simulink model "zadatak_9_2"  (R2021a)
settings: Solver=VariableStepAuto  StartTime=0.0  StopTime=5/50  RelTol=1e-3
libraries: spsGroundLib x2, spsVoltageMeasurementLib x2, spsBoostConverterLib x1, spsDCVoltageSourceLib x1, spsSeriesRLCLoadLib x1, spspowerguiLib x1

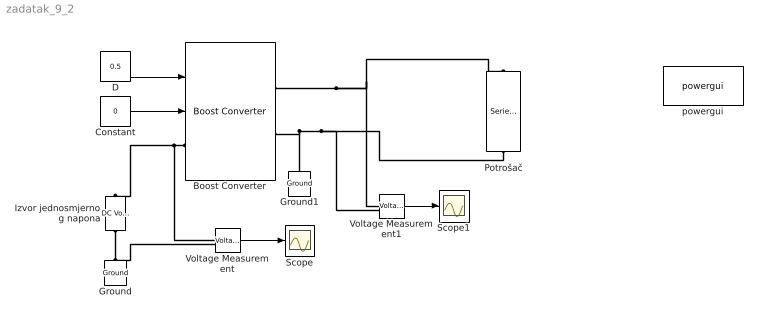
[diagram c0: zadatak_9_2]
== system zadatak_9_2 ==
  Boost Converter : spsBoostConverterLib/Boost Converter  ModelType=Average model (D-controlled)  Ron=1e-3  Rs=1e6  Cs=inf  Vforward=[0,0]  Ron_Diode=1e-3  Rs_Diode=1e6  Cs_Diode=inf  Vf_Diode=1e-3  Rs_CurrentSource=inf
  Constant : Constant  Value=0
  D : Constant  Value=0.5
  Ground : spsGroundLib/Ground  LConnTagsString=a
  Ground1 : spsGroundLib/Ground  LConnTagsString=a
  Izvor jednosmjernog napona : spsDCVoltageSourceLib/DC Voltage Source  Amplitude=50  Measurements=None
  Potrošač : spsSeriesRLCLoadLib/Series RLC Load  LConnTagsString=a  RConnTagsString=__new0  NominalVoltage=50/0.5  NominalFrequency=50  ActivePower=1500  InductivePower=0  CapacitivePower=0  Setx0=off  InitialVoltage=0  SetiL0=off  InitialCurrent=0  Measurements=None  LoadType=constant Z
  Scope : Scope
  Scope1 : Scope
  Voltage Measurement : spsVoltageMeasurementLib/Voltage Measurement  PhasorSimulation=off  OutputType=Complex  PSBequivalent=0
  Voltage Measurement1 : spsVoltageMeasurementLib/Voltage Measurement  PhasorSimulation=off  OutputType=Complex  PSBequivalent=0
  powergui : spspowerguiLib/powergui  Priority=1  SimulationMode=Continuous  SampleTime=50e-6  frequency=60  Iterations=50  frequencyindice=0  Pbase=100e6  ErrMax=1e-4  UnitsV=kV  UnitsW=MW  buscounter=0  FunctionMessages=off  echomessages=off  EnableUseOfTLC=off  CurrentSourceSwitches=off  DisableSnubberDevices=off  DisableRonSwitches=off  DisableVfSwitches=off  DisplayEquations=off  AutomaticDiscreteSolvers=off  SolverType=Tustin/Backward Euler (TBE)  Interpol=off  ExternalGateDelay=off  methode=off  Ts=100  x0status=blocks  SPID=on  SwTol=0  HookPort=off  NonlinearTolerance=1e-4  nMaxIteration=100  ContinueOnMaxIteration=off  RestoreLinks=warning  ResistiveCurrentMeasurement=off  Frange=[0:2:500]  Ylog=off  Xlog=on  ShowGrid=off  save=off  variable=ZData  structure=0  ZoomFFT=off  StartTime=0.0  cycles=1  DisplayStyle=1  fundamental=60  FreqAxis=off  MaxFrequency=1000  frequencyindicesteady=1  RmsSteady=1  display=off
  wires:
  D/1 -> Boost Converter/1
  Constant/1 -> Boost Converter/2
  Voltage Measurement/1 -> Scope/1
  Voltage Measurement1/1 -> Scope1/1
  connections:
  Ground/LConn1 -- Voltage Measurement/LConn2 -- Izvor jednosmjernog napona/LConn1
  Boost Converter/LConn1 -- Voltage Measurement/LConn1 -- Izvor jednosmjernog napona/RConn1
  Boost Converter/RConn1 -- Voltage Measurement1/LConn1 -- Potrošač/LConn1
  Potrošač/RConn1 -- Voltage Measurement1/LConn2 -- Ground1/LConn1 -- Boost Converter/RConn2
